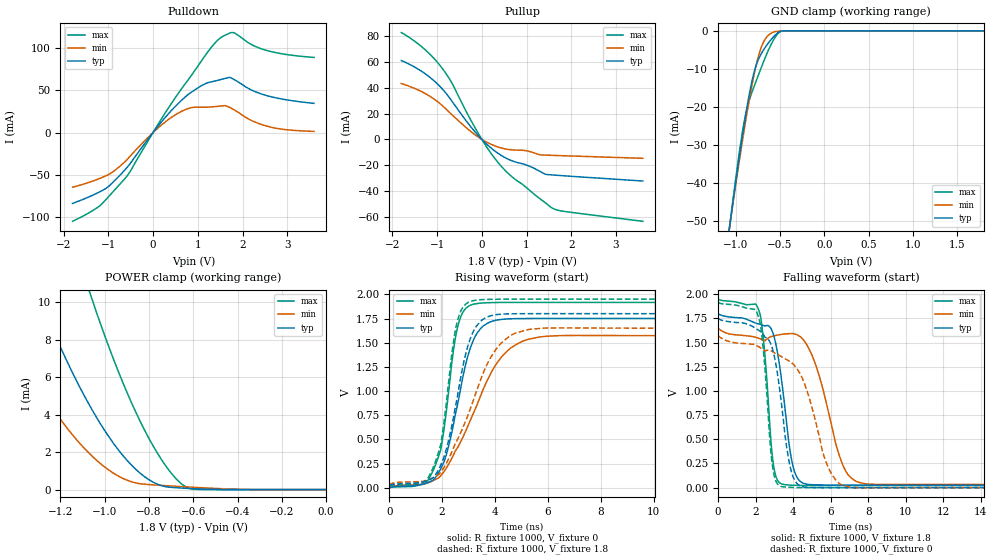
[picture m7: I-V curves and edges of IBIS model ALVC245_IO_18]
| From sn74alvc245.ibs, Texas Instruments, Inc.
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[Model]   ALVC245_IO_18
Model_type  I/O
Vinl=0.5775
Vinh=1.2675
Enable   Active-Low
Vref =   0
Rref =   1000
Cref =   30p
Vmeas =   0.9
| variable   typ   min   max
C_comp   8.58pF   8.27pF   9.31pF
| C_pullup   10.93pF   8.29pF   13.69pF
| C_pulldown   15.00pF   8.76pF   23.41pF
| C_tri-state   8.58pF   8.27pF   9.31pF
[Temperature Range]   40   100   -40
| Ambient temperature   25   85   -40
[Voltage range]   1.8   1.65   1.95
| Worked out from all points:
|   slope of the pulldown table from 0 to 0.27 V, typ, clamps not added: 15.3 ohm
|   slope of the pullup table from 0 to 0.27 V, typ, clamps not added: 31.8 ohm
|   GND clamp passes 1 mA (typ) near -0.55 V on its own axis
|   POWER clamp passes 1 mA (typ) near -0.85 V on its own axis
|   rising waveform, R_fixture 1000, V_fixture 0: 20-80 % time 850ps typ, 1.62ns min, 556ps max; typ from 0 V to 1.75 V
|   falling waveform, R_fixture 1000, V_fixture 1.8: 20-80 % time 717ps typ, 1.33ns min, 448ps max; typ from 1.8 V to 0.026 V
|   rising waveform, R_fixture 1000, V_fixture 1.8: 20-80 % time 812ps typ, 1.45ns min, 555ps max; typ from 0.026 V to 1.8 V
|   falling waveform, R_fixture 1000, V_fixture 0: 20-80 % time 766ps typ, 1.57ns min, 452ps max; typ from 1.75 V to 0 V
[GND Clamp]
| ALVC245_IO_18
|   Voltage   I(typ)   I(min)   I(max)
-1.8V     -189.6mA   -180.2mA   -200.4mA
-1.07V    -51.77mA   -51.73mA   -51.66mA
-1.05V    -48.29mA   -48.49mA   -47.93mA
-970mV    -34.83mA   -35.87mA   -33.75mA
-915mV    -26.17mA   -27.62mA   -25.32mA
-870mV    -19.69mA   -21.24mA   -20.16mA
-815mV    -13.02mA   -14.11mA   -16.05mA
-770mV    -9.128mA   -9.109mA   -13.24mA
-710mV    -5.956mA   -4.23mA    -9.579mA
-595mV    -2.136mA   -575.9uA   -3.319mA
-475mV    -22.44uA   -72.77uA   -18.11uA
1.8V      62.68pA    15.05nA    10.36pA
[POWER Clamp]
| ALVC245_IO_18
|   Voltage   I(typ)   I(min)   I(max)
-1.8V     27.95mA    17.5mA     45.21mA
-1.53V    17.77mA    10.42mA    30.77mA
-1.3V     10.36mA    5.491mA    19.85mA
-1.17V    6.843mA    3.283mA    14.39mA
-1.06V    4.323mA    1.821mA    10.26mA
-990mV    2.975mA    1.115mA    7.897mA
-915mV    1.779mA    583.1uA    5.625mA
-835mV    826.5uA    303.9uA    3.528mA
-755mV    257.5uA    232.7uA    1.813mA
-685mV    108.7uA    181.3uA    674.9uA
-630mV    68.37uA    143.7uA    124.3uA
-16.28fV  62.68pA    441.1pA    11.57pA
[Pulldown]
| ALVC245_IO_18
|   Voltage   I(typ)   I(min)   I(max)
-1.8V     -83.87mA   -64.71mA   -105mA
-1.195V   -70.25mA   -54.39mA   -86.97mA
-980mV    -63.08mA   -49.25mA   -75.07mA
-605mV    -42.71mA   -33.22mA   -52.94mA
70mV      4.77mA     3.453mA    6.125mA
555mV     34.03mA    22.77mA    45.71mA
1.09V     55.68mA    29.91mA    85.43mA
1.525V    62.86mA    31.48mA    112.8mA
1.805V    62.94mA    27.18mA    118.1mA
2.205V    50.22mA    14.19mA    104mA
2.565V    43.4mA     7.307mA    96.81mA
3.6V      34.57mA    1.347mA    88.92mA
[Pullup]
| ALVC245_IO_18
|   Voltage   I(typ)   I(min)   I(max)
-1.8V     61.12mA    43.3mA     82.82mA
-1.29V    51.46mA    35.99mA    70.21mA
-870mV    38.57mA    25.77mA    54.36mA
-660mV    29.2mA     18.85mA    43.11mA
-200mV    7.791mA    4.825mA    11.98mA
240mV     -7.675mA   -4.32mA    -12.5mA
605mV     -15.61mA   -7.888mA   -26.92mA
970mV     -19.57mA   -8.672mA   -36.62mA
1.255V    -24mA      -11.53mA   -44.89mA
1.425V    -27.07mA   -12.21mA   -49.36mA
1.73V     -27.99mA   -12.59mA   -55.2mA
3.6V      -32.32mA   -14.7mA    -63.54mA
[Ramp]
| ALVC245_IO_18
| variable   typ   min   max
dV/dt_r   1.05/8.68E-10   0.94/1.68E-09   1.15/5.62E-10
dV/dt_f   1.06/7.28E-10   0.97/1.37E-09   1.16/4.73E-10
R_load = 1000
[Rising Waveform]
| ALVC245_IO_18
R_fixture =   1000
C_fixture =   0
L_fixture =   0
V_fixture =   0
V_fixture_min = 0
V_fixture_max = 0
|   Time   V(typ)   V(min)   V(max)
0s        267.6pV    3.892nV    40.96pV
1.63ns    76.02mV    69.74mV    161.6mV
1.955ns   201.2mV    128.3mV    405.9mV
2.425ns   650.2mV    338.4mV    1.413V
2.615ns   903.5mV    430.9mV    1.691V
2.96ns    1.349V     631mV      1.869V
3.31ns    1.593V     851.8mV    1.904V
4.49ns    1.746V     1.421V     1.916V
6.255ns   1.751V     1.571V     1.916V
50ns      1.75V      1.573V     1.916V
[Falling Waveform]
| ALVC245_IO_18
R_fixture =   1000
C_fixture =   0
L_fixture =   0
V_fixture =   1.8
V_fixture_min = 1.65
V_fixture_max = 1.95
|   Time   V(typ)   V(min)   V(max)
0s        1.8V       1.65V      1.95V
2.18ns    1.692V     1.544V     1.831V
2.45ns    1.675V     1.524V     1.472V
2.945ns   1.588V     1.569V     246.4mV
3.49ns    949mV      1.588V     33.36mV
4.3ns     80.28mV    1.572V     23.1mV
5.225ns   28.88mV    1.258V     21.93mV
6.7ns     25.94mV    210.8mV    21.88mV
7.845ns   25.83mV    40.25mV    21.9mV
50ns      25.82mV    32.4mV     21.92mV
[Rising Waveform]
| ALVC245_IO_18
R_fixture =   1000
C_fixture =   0
L_fixture =   0
V_fixture =   1.8
V_fixture_min = 1.65
V_fixture_max = 1.95
|   Time   V(typ)   V(min)   V(max)
0s        25.82mV    32.4mV     21.91mV
1.585ns   93.18mV    95.37mV    163.3mV
1.95ns    237.9mV    164mV      451mV
2.385ns   667.3mV    382.4mV    1.423V
2.58ns    945.8mV    499.6mV    1.726V
2.925ns   1.42V      714.9mV    1.905V
3.285ns   1.666V     987.8mV    1.94V
4.245ns   1.795V     1.498V     1.95V
5.835ns   1.8V       1.65V      1.95V
50ns      1.8V       1.65V      1.95V
[Falling Waveform]
| ALVC245_IO_18
R_fixture =   1000
C_fixture =   0
L_fixture =   0
V_fixture =   0
V_fixture_min = 0
V_fixture_max = 0
|   Time   V(typ)   V(min)   V(max)
0s        1.75V      1.573V     1.916V
2.11ns    1.634V     1.464V     1.793V
2.405ns   1.585V     1.427V     1.442V
2.89ns    1.442V     1.409V     237.9mV
3.385ns   861.2mV    1.355V     10.9mV
3.815ns   240.1mV    1.305V     3.578mV
4.205ns   43.45mV    1.23V      1.257mV
5.885ns   247.7uV    204.7mV    -62.38uV
7.08ns    -3.85uV    1.874mV    -20.46uV
50ns      1.257uV    -516.3nV   363.1nV
